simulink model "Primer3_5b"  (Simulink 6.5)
settings: Solver=ode23t  SolverMode=SingleTasking  StartTime=0.0  StopTime=0  RelTol=1e-3  AbsTol=1e-6
undefined symbols (not defined in the file or in its folder): Phasor, powergui, steady, ZData
libraries: powerlib x20

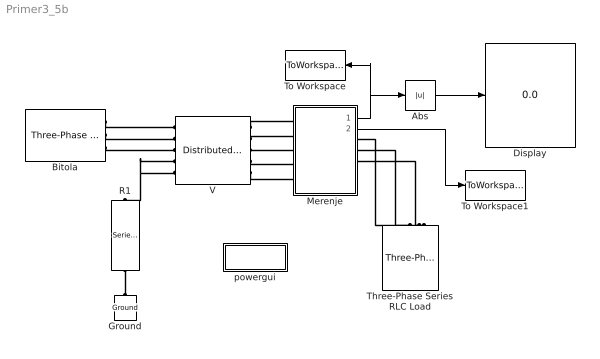
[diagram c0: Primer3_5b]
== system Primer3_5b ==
  Abs : Abs  SampleTime=-1
  Bitola : powerlib/Electrical Sources/Three-Phase Source  DialogController=PMDialogs.PMDefaultMaskDlg  SystemSampleTime=-1  Voltage=410e3  PhaseAngle=0  Frequency=50  InternalConnection=Yg  SpecifyImpedance=on  Resistance=0.8929  Inductance=16.58e-3  ShortCircuitLevel=sqrt(3)*400e3*16e3  BaseVoltage=400e3  XRratio=10
  Display : Display
  Ground : powerlib/Elements/Ground  Orientation=down  DialogController=PMDialogs.PMDefaultMaskDlg  PhysicalDomain=powersysdomain  SubClassName=unknown  LeftPortType=p1  RightPortType=p1  LConnTagsString=a
  Merenje : Subsystem
  R1 : powerlib/Elements/Series RLC Branch  Orientation=down  DialogController=PMDialogs.PMDefaultMaskDlg  PhysicalDomain=powersysdomain  SubClassName=unknown  LeftPortType=p1  RightPortType=p1  LConnTagsString=__new0  RConnTagsString=__new0  BranchType=R  Resistance=0.5  Inductance=1e-3  SetiL0=off  InitialCurrent=0  Capacitance=1e-6  Setx0=off  InitialVoltage=0  Measurements=None
  Three-Phase Series RLC Load : powerlib/Elements/Three-Phase Series RLC Load  Orientation=down  DialogController=PMDialogs.PMDefaultMaskDlg  PhysicalDomain=powersysdomain  SubClassName=unknown  LeftPortType=p1  RightPortType=p1  LConnTagsString=A|B|C  Configuration=Y (grounded)  NominalVoltage=400e3  NominalFrequency=50  ActivePower=1000e6  InductivePower=0  CapacitivePower=0  Measurements=None
  To Workspace : ToWorkspace  VariableName=napon  SampleTime=-1  SaveFormat=Array
  To Workspace1 : ToWorkspace  VariableName=struja  SampleTime=-1  SaveFormat=Array
  V : powerlib/Elements/Distributed Parameters Line  DialogController=PMDialogs.PMDefaultMaskDlg  SystemSampleTime=-1  Phases=5  Frequency=50  Resistance=[0.077552 0.048545 0.048526 0.04828 0.048266;0.048545 0.077556 0.048545 0.04828 0.04828;0.048526 0.048545 0.077552 0.048266 0.04828;0.04828 0.04828 0.048266 0.66802 0.048008;0.048266 0.04828 0.04828 0.048008 0.66802]  Inductance=[0.0019739 0.0010122 0.00087354 0.0010299 0.00089553;0.0010122 0.0019739 0.0010122 0.0010089 0.0010089;0.00087354 0.0010122 0.0019739 0.00089553 0.0010299;0.0010299 0.0010089 0.00089553 0.0024807 0.00097794;0.00089553 0.0010089 0.0010299 0.00097794 0.0024807]  Capacitance=[1.0643e-008 -1.3918e-009 -3.4639e-010 -1.2909e-009 -4.2739e-010;-1.3918e-009 1.0936e-008 -1.3918e-009 -1.0228e-009 -1.0228e-009;-3.4639e-010 -1.3918e-009 1.0643e-008 -4.2739e-010 -1.2909e-009;-1.2909e-009 -1.0228e-009 -4.2739e-010 7.0383e-009 -7.334e-010;-4.2739e-010 -1.0228e-009 -1.2909e-009 -7.334e-010 7.0383e-009]  Length=113.5  x1=[0 14893.3498499213 -265760.761035288 -299224.975732838 4130.99388800946 -31361.7072191121;0.000130826521382094 15545.0371505606 -253291.346753453 -309924.773047741 4268.81351487322 -29883.5992320992;0.000261653042764188 16170.4688503813 -240394.122848089 -320101.106761618 4399.4231066287 -28355.0177824076;0.000392479564146282 16768.588593912 -227090.872757808 -329736.789025177 4522.60206339754 -2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  x2=[0 15549.9774599514 -315188.676611296 -232878.503981479 4157.03637271974 -31555.2307335966;0.000130826521382094 16314.5072713454 -305970.85161103 -245418.721074121 4284.95786372597 -30126.0615615285;0.000261653042764188 17051.4818452498 -296236.241191456 -257544.425424753 4405.64205178435 -28646.0094073914;0.000392479564146282 17759.6564300416 -286001.287130284 -269235.136692932 4518.8851010445 -2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  x3=[0 0.574706429682641 1030.06047446506 475.890778824079 11.968119892819 -63.0373443931273;0.000130826521382094 1.64732304613298 1007.12038908227 509.542497025588 12.2297244722786 -60.6335759411517;0.000261653042764188 2.7171573304538 982.479275219727 542.333596865596 12.4706730210864 -58.1273972504169;0.000392479564146282 3.78240233026289 956.178751771165 574.208694106714 12.690558576631 -55.523041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  x4=[0 29.6363655537887 -2941.11159730504 -2301.04819532639 6.69129238800283 -75.3755777123358;0.000130826521382094 30.3109413846056 -2855.07958853036 -2425.00561429881 7.11101718177682 -72.12817279352;0.000261653042764188 30.934321970939 -2764.22534425662 -2544.86719362961 7.51873145240248 -68.7589432374072;0.000392479564146282 31.5054544216524 -2668.7023174957 -2660.4304868563 7.91374656960934 -65.2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  x5=0.00065413260691047  Measurements=None
  powergui : Subsystem  AncestorBlock=powerlib/powergui  InitFcn=powergui( 'InitFcn_Callback' , gcb , 0 , [ ] );  mask(PSB option menu block){SimulationMode=Phasor, SampleTime=50e-6, echomessages=off, RestoreLinks=warning, x0status=steady, Frange=[0:2:500], Ylog=off, Xlog=on, ShowGrid=off, save=off, variable=ZData, structure=, ZoomFFT=on, StartTime=0.0, cycles=1, DisplayStyle=1, fundamental=60, FreqAxis=off, MaxFrequency=1000, frequencyindice=50, frequencyindicesteady=1, RmsSteady=2, display=off, Ts=0, frequency=50, methode=off, HookPort=off, Interpol=off}
      mask prompts: SimulationMode "Simulation mode"; SampleTime "Sample time Ts (when simulation mode is Discrete) (s)"; echomessages "Echo  Messages"; RestoreLinks "Restore disabled links"; x0status "Initial electrical states status"; Frange "Impedance tool: Frequency Range"; Ylog "Impedance tool: Log impedance"; Xlog "Impedance tool: log Frequency"; ShowGrid "Impedance tool: grid"; save "Impedance tool: Save Data To Workspace"; variable "Impedance tool: Variable Name"; structure "Structure Name (PSBFFTSCOPE)"; ZoomFFT "ZoomFFT (PSBFFTSCOPE)"; StartTime "Start Time (PSBFFTSCOPE)"; cycles "Cycles (PSBFFTSCOPE)"; DisplayStyle "Display style (PSBFFTSCOPE)"; fundamental "Fundamental (PSBFFTSCOPE)"; FreqAxis "Frequency Axis (PSBFFTSCOPE)"; MaxFrequency "Max Frequency (PSBFFTSCOPE)"; frequencyindice "Load flow frequency (Hz)"; frequencyindicesteady "Frequency indice (STEADYSTATE)"; RmsSteady "RMS display (STEADYSTATE)"; display "Display Results"; Ts "OBSOLETE 1"; frequency "Phasor frequency (Hz)"; methode "Phasor simulation"; HookPort "Hook port"; Interpol "Interpolate"
      mask init:
      | powerlibroot = which('powersysdomain');
      | PSBroot = powerlibroot(1:end-16);
      | %
      | switch SimulationMode
      | 	case 1
      | 		message=sprintf('Continuous');
      | 	case 2
      |         SampleTimeeval=evalin('base',SampleTime,'NaN');
      |         if isnan(SampleTimeeval)
      |             message=sprintf('Warning !!,\nUndefined sample time');
      |         else
      |             message=sprintf('Discrete,\nTs = %.4g s.',SampleTimeeval);
      |         end
      | 	case 3
      | 		message=sprintf('Phasors');
      | end
      | if strcmp(bdroot,'powerlib')
      |   message='powergui';
      | end
      | power_initmask();
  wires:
  Merenje/1(U) -> Abs/1, To Workspace/1
  Abs/1 -> Display/1
  Merenje/2(I) -> To Workspace1/1
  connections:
  Ground/LConn1 -- R1/RConn1
  V/RConn1 -- Merenje/LConn1
  V/RConn2 -- Merenje/LConn2
  V/RConn3 -- Merenje/LConn3
  V/RConn4 -- Merenje/LConn4
  V/RConn5 -- Merenje/LConn5
  Merenje/RConn1 -- Three-Phase Series RLC Load/LConn1
  Merenje/RConn2 -- Three-Phase Series RLC Load/LConn2
  Merenje/RConn3 -- Three-Phase Series RLC Load/LConn3
  Bitola/RConn1 -- V/LConn1
  Bitola/RConn2 -- V/LConn2
  Bitola/RConn3 -- V/LConn3
  V/LConn5 -- R1/LConn1 -- V/LConn4

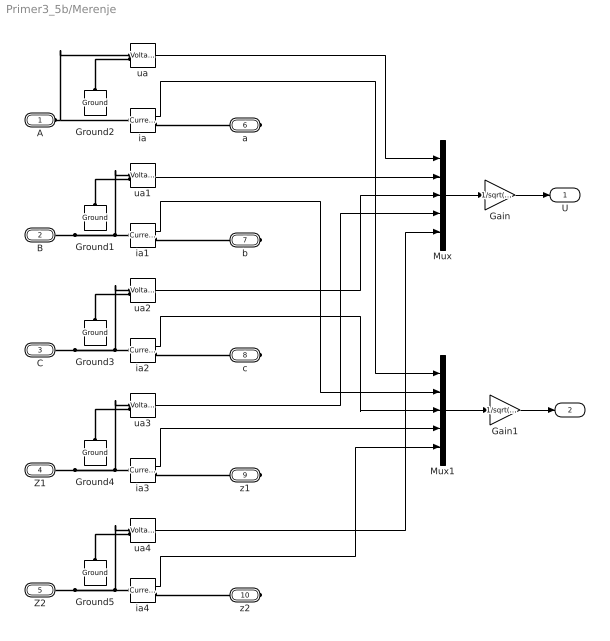
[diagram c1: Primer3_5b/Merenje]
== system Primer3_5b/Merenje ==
  Gain : Gain  Gain=1/sqrt(2)
  Gain1 : Gain  Gain=1/sqrt(2)
  Ground{1..5} (5 alike) : powerlib/Elements/Ground  Orientation=down  DialogController=PMDialogs.PMDefaultMaskDlg  PhysicalDomain=powersysdomain  SubClassName=unknown  LeftPortType=p1  RightPortType=p1  LConnTagsString=a
  Mux : Mux  Inputs=5
  Mux1 : Mux  Inputs=5
  ia{,1..4} (5 alike) : powerlib/Measurements/Current Measurement  DialogController=PMDialogs.PMDefaultMaskDlg  SystemSampleTime=-1  PhasorSimulation=on  OutputType=Complex  PSBequivalent=0
  ua{,1..4} (5 alike) : powerlib/Measurements/Voltage Measurement  DialogController=PMDialogs.PMDefaultMaskDlg  SystemSampleTime=-1  PhasorSimulation=on  OutputType=Complex  PSBequivalent=0
  A : PMIOPort  Port=1  Side=Left
  B : PMIOPort  Port=2  Side=Left
  C : PMIOPort  Port=3  Side=Left
  Z1 : PMIOPort  Port=4  Side=Left
  Z2 : PMIOPort  Port=5  Side=Left
  a : PMIOPort  Orientation=left  Port=6  Side=Right
  b : PMIOPort  Orientation=left  Port=7  Side=Right
  c : PMIOPort  Orientation=left  Port=8  Side=Right
  z1 : PMIOPort  Orientation=left  Port=9  Side=Right
  z2 : PMIOPort  Orientation=left  Port=10  Side=Right
  U : Outport
  I : Outport  Port=2
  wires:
  ua/1 -> Mux/1
  ia/1 -> Mux1/1
  ua1/1 -> Mux/2
  ia1/1 -> Mux1/2
  ua2/1 -> Mux/3
  ia2/1 -> Mux1/3
  ua3/1 -> Mux/4
  ia3/1 -> Mux1/4
  ua4/1 -> Mux/5
  ia4/1 -> Mux1/5
  Mux/1 -> Gain/1
  Gain/1 -> U/1
  Mux1/1 -> Gain1/1
  Gain1/1 -> I/1
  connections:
  A/RConn1 -- ia/LConn1 -- ua/LConn1
  ia/RConn1 -- a/RConn1
  Ground2/LConn1 -- ua/LConn2
  ia1/LConn1 -- B/RConn1 -- ua1/LConn1
  Ground1/LConn1 -- ua1/LConn2
  ia1/RConn1 -- b/RConn1
  ia2/LConn1 -- ua2/LConn1 -- C/RConn1
  ia2/RConn1 -- c/RConn1
  Ground3/LConn1 -- ua2/LConn2
  ia3/LConn1 -- Z1/RConn1 -- ua3/LConn1
  Ground4/LConn1 -- ua3/LConn2
  ia3/RConn1 -- z1/RConn1
  ia4/LConn1 -- ua4/LConn1 -- Z2/RConn1
  Ground5/LConn1 -- ua4/LConn2
  ia4/RConn1 -- z2/RConn1

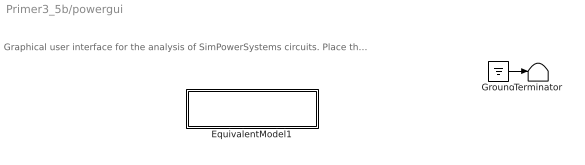
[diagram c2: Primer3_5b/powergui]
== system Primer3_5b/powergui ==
  note: Graphical user interface for the analysis of SimPowerSystems circuits. Place the Powergui block in the top-level of your model and double-click on it to open the GUI.
  EquivalentModel1 : Subsystem
  Ground : Ground
  Terminator : Terminator
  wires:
  Ground/1 -> Terminator/1

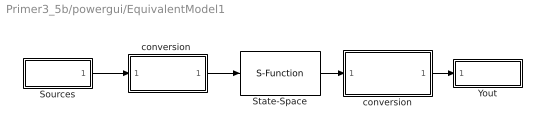
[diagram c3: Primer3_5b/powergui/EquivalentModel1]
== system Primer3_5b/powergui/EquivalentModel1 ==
  Sources : Subsystem
  State-Space : S-Function  FunctionName=sfun_psbdqc  Parameters=H, Rswitch,InputsNonZero
  Yout : Subsystem
  conversion : Subsystem
  "conversion " : Subsystem
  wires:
  State-Space/1 -> conversion/1(Yout)
  conversion/1(Complex) -> Yout/1(v,i)
  "conversion "/1(u) -> State-Space/1
  Sources/1(u) -> "conversion "/1(Complex)

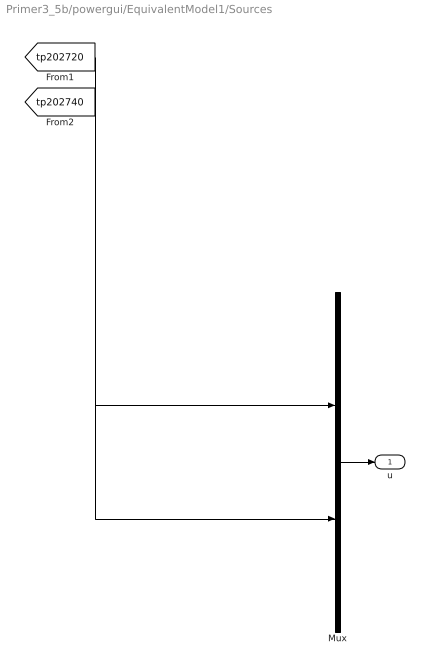
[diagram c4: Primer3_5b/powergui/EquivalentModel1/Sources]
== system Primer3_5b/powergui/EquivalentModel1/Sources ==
  Mux : Mux  Inputs=[10 3]
  u : Outport
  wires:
  Mux/1 -> u/1
  [tp202720] -> Mux/1
  [tp202740] -> Mux/2

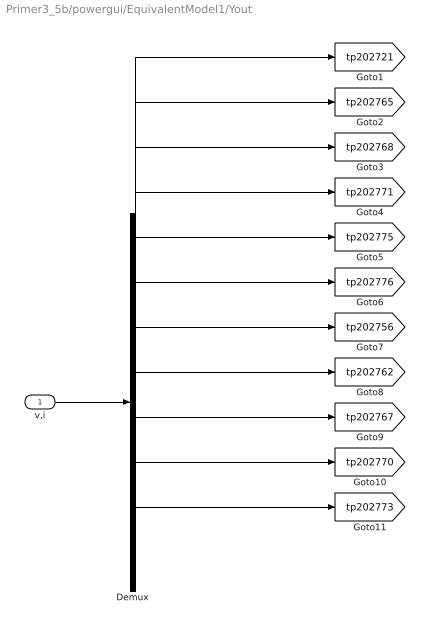
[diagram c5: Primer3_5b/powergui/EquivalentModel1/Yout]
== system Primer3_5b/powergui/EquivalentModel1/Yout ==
  v,i : Inport
  Demux : Demux  Outputs=[10 1 1 1 1 1 1 1 1 1 1]
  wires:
  v,i/1 -> Demux/1
  Demux/1 -> [tp202721]
  Demux/2 -> [tp202765]
  Demux/3 -> [tp202768]
  Demux/4 -> [tp202771]
  Demux/5 -> [tp202775]
  Demux/6 -> [tp202776]
  Demux/7 -> [tp202756]
  Demux/8 -> [tp202762]
  Demux/9 -> [tp202767]
  Demux/10 -> [tp202770]
  Demux/11 -> [tp202773]

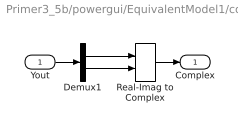
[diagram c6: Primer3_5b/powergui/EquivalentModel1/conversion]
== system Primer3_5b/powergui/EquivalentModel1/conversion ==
  Yout : Inport
  Demux1 : Demux  Outputs=2
  Real-Imag to Complex : RealImagToComplex
  Complex : Outport
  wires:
  Demux1/1 -> Real-Imag to Complex/1
  Demux1/2 -> Real-Imag to Complex/2
  Real-Imag to Complex/1 -> Complex/1
  Yout/1 -> Demux1/1

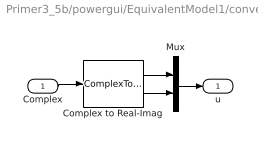
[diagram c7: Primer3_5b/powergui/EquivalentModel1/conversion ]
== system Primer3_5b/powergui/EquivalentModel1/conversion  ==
  Complex : Inport
  Complex to Real-Imag : ComplexToRealImag
  Mux : Mux  Inputs=2
  u : Outport
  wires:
  Complex to Real-Imag/1 -> Mux/1
  Complex to Real-Imag/2 -> Mux/2
  Complex/1 -> Complex to Real-Imag/1
  Mux/1 -> u/1
